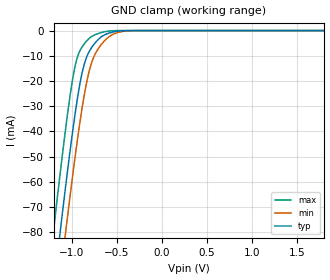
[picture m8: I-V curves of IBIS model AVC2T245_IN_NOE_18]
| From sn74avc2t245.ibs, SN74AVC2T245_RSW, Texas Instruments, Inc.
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[Model]   AVC2T245_IN_NOE_18
Model_type  Input
Vinl=0.5775
Vinh=1.2675
| variable   typ   min   max
C_comp   2.78pF   2.15pF   3.16pF
[Temperature Range]   40   100   -40
| Ambient temperature   25   85   -40
[Voltage range]   1.8   1.65   1.95
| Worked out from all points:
|   GND clamp passes 1 mA (typ) near -0.58 V on its own axis
[GND Clamp]
| AVC2T245_IN_NOE_18
|   Voltage   I(typ)   I(min)   I(max)
-4.6V     -1.266A    -1.277A    -1.254A
-1.2V     -102.6mA   -121mA     -79.39mA
-1.135V   -82.53mA   -100.9mA   -59.27mA
-1.115V   -76.45mA   -94.78mA   -53.25mA
-1.065V   -61.6mA    -79.78mA   -38.73mA
-960mV    -32.94mA   -49.96mA   -14.03mA
-905mV    -20.72mA   -35.89mA   -7.898mA
-860mV    -13.49mA   -25.81mA   -5.335mA
-760mV    -5.854mA   -11.09mA   -2.009mA
-585mV    -1.007mA   -2.481mA   -186.3uA
-310mV    -2.903uA   -30.35uA   -13.82nA
1.8V      127.8pA    12.94nA    23.41pA
